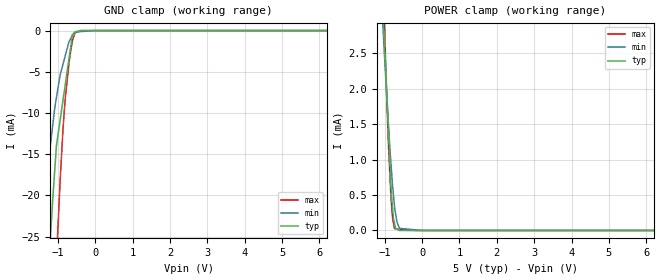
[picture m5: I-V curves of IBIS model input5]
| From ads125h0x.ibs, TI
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|   input5 Model
[Model]   input5
Model_type   Input
Vinl = 1.5
Vinh = 3.5
|   typ   min   max
C_comp   2.088pF   1.785pF   2.310pF
|  Where Nom  PVT is Nominal Process,   5V,  27C
|   Fast PVT is Strong Process,   5.25V, -40C
|   Slow PVT is Weak Process,   2.7V, 135C
[Model spec]
|subparameter
Vinl   1.500   0.810   1.575
Vinh   3.500   1.890   3.675
[Voltage Range]   5   2.7   5.25
|Junction Temperature
[Temperature Range]   27   135   -40
[Power Clamp Reference]   5   2.7   5.25
[GND Clamp Reference]   0   0   0
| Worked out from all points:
|   GND clamp passes 1 mA (typ) near -0.62 V on its own axis
|   POWER clamp passes 1 mA (typ) near -0.86 V on its own axis
[GND Clamp]
|   Voltage   I(typ)   I(min)   I(max)
-5V       -411.9mA   -286.8mA   -505.9mA
-1.431V   -44.3mA    -24.61mA   -72.57mA
-1.25V    -29.13mA   -15.99mA   -51.34mA
-1.136V   -20.62mA   -11.56mA   -38.61mA
-1.02V    -13.49mA   -7.699mA   -26.27mA
-940.2mV  -10.99mA   -5.469mA   -18.67mA
-859.7mV  -8.464mA   -4.084mA   -11.98mA
-791.3mV  -6.315mA   -2.908mA   -7.918mA
-691.6mV  -3.18mA    -1.281mA   -3.661mA
-607.2mV  -526.9uA   -539.8uA   -1.237mA
-552.1mV  -174.7uA   -334.3uA   -465.3uA
10V       0A         0A         0A
[POWER Clamp]
|   Voltage   I(typ)   I(min)   I(max)
-5V       83.73mA    65.22mA    101.9mA
-1.066V   3.518mA    3.079mA    4.189mA
-1.036V   3.031mA    2.785mA    3.575mA
-1.003V   2.647mA    2.462mA    2.902mA
-950.8mV  2.04mA     1.964mA    1.972mA
-895.1mV  1.391mA    1.477mA    1.176mA
-821.5mV  531.1uA    879.8uA    407.7uA
-785.2mV  302.4uA    615.8uA    163.3uA
-736.6mV  104.6uA    351.5uA    25.62uA
-671.1mV  17.6uA     123.9uA    22.61uA
-607.2mV  809.2nA    34.72uA    19.67uA
10V       0A         0A         0A
